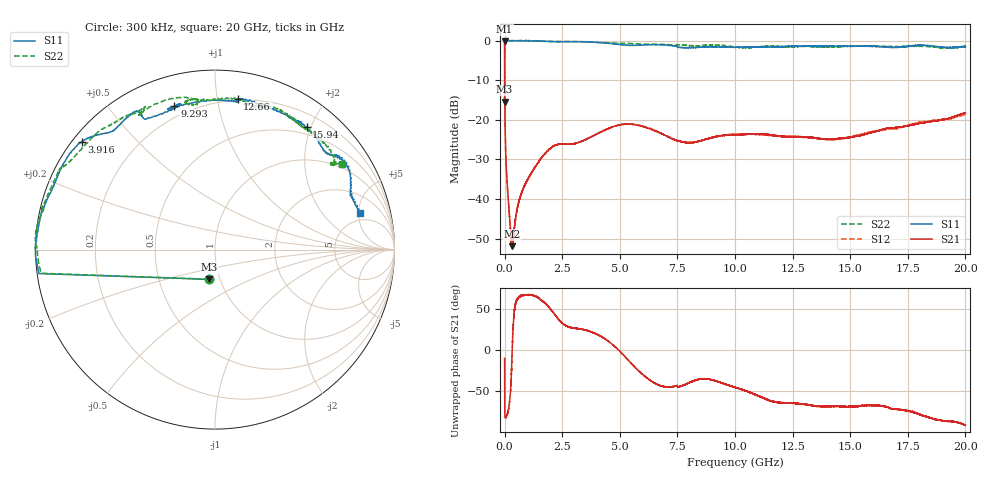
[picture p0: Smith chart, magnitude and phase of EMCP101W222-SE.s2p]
!EMCP101W222
!Johanson Technology Inc.
!www.johansontechnology.com
!Test Board Conditions:
!Substrate Type  RO4350B
!Substrate Thickness  10 mil
!Substrate Dk  3.66
!TL Type: GCPW
!TL Trace Width  20 mil
!TL Gap  10 mil
!PART MODE SINGLE ENDED (AKA BYPASS)
!DUT TOPOLOGY	SERIES-SHUNT
# MHz S  dB  R 50
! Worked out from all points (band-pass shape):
!   20001 points, 300 kHz to 20 GHz, reference 50 ohm
!   highest |S21| = -0.14 dB at 300 kHz (marker M1); lowest = -51.9 dB at 324.3 MHz (marker M2)
!   |S21| within 3 dB of the highest: start of sweep to 1.789 MHz
!   lowest |S11| = -15.4 dB at 300 kHz (marker M3), VSWR 1.41, Z = 44.4 - j15.2 ohm
!   |S11| at or under -10 dB: start of sweep to 801.5 kHz
!   |S22| runs from -15.5 to 0.0 dB; largest |S21 - S12| = 0.0067
!   S11 on the Smith chart (normalised r, x): 300 kHz: 0.89, -0.30; 3.916 GHz: 0.03, +0.35; 9.293 GHz: 0.14, +0.75; 12.66 GHz: 0.19, +1.14; 15.94 GHz: 0.39, +1.94; 20 GHz: 3.85, +5.20
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0.3  -15.44 -101.1  -0.14 -9.7  -0.14 -9.9  -15.50 -100.7
101.298  0.01 -179.6  -35.15 -78.7  -35.09 -78.9  -0.09 -179.4
127.298  0.02 179.9  -37.51 -76.6  -37.47 -76.6  -0.09 -179.7
238.296  0.00 178.7  -46.32 -55.4  -46.37 -56.1  -0.06 179.3
324.295  -0.01 177.6  -51.88 -4.1  -51.33 -5.4  -0.03 178.9
769.288  -0.06 173.6  -37.94 65.8  -37.95 66.4  0.03 175.5
1600.276  -0.15 166.8  -29.57 60.8  -29.55 60.9  -0.13 164.5
2205.267  -0.27 160.7  -26.40 42.4  -26.35 42.2  -0.22 157.3
3334.25  -0.27 147.2  -25.43 25.7  -25.45 25.7  -0.26 152.0
3916.241  -0.41 140.9  -23.83 20.5  -23.82 20.5  -0.45 149.6
5258.221  -1.13 131.8  -21.06 -8.7  -21.11 -8.4  -0.69 135.3
6667.2  -1.02 120.3  -23.11 -41.8  -23.03 -42.2  -0.95 125.4
7954.181  -1.79 110.7  -25.77 -40.1  -25.71 -40.1  -1.24 118.2
8630.171  -1.62 103.5  -25.07 -34.7  -25.09 -35.1  -1.23 117.6
9293.161  -1.60 105.7  -24.08 -38.6  -24.14 -37.9  -1.19 105.5
10000.15  -1.69 107.8  -23.77 -44.9  -23.61 -44.8  -1.61 96.7
11429.13  -1.58 82.9  -23.70 -60.1  -23.84 -59.8  -1.45 100.2
12659.11  -1.42 81.5  -24.27 -64.4  -24.19 -64.6  -1.47 87.4
13334.1  -1.45 75.8  -24.46 -67.0  -24.44 -67.4  -1.50 79.6
15942.06  -1.39 53.1  -23.20 -67.0  -23.01 -68.0  -1.44 59.2
16667.05  -1.68 43.9  -22.05 -69.5  -22.31 -70.1  -1.49 56.5
20000  -1.58 14.3  -18.24 -91.2  -18.56 -89.5  -1.37 33.8
